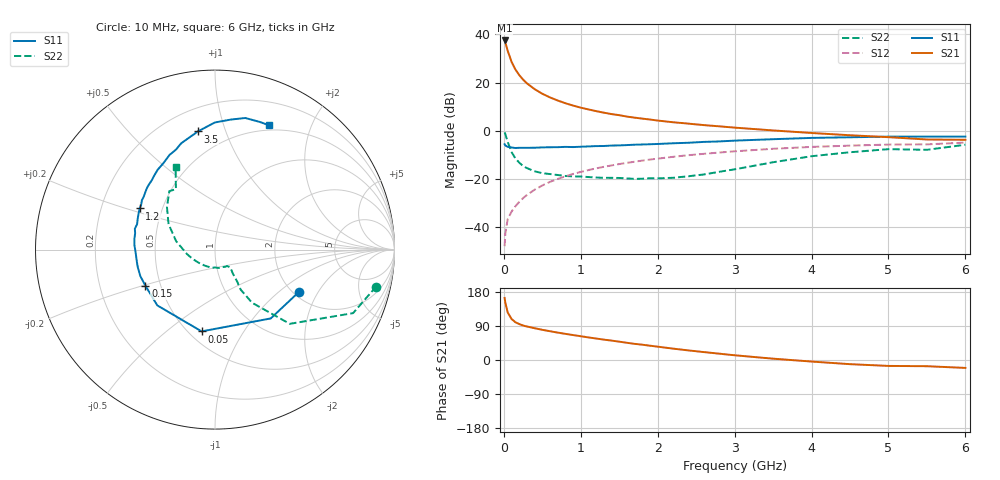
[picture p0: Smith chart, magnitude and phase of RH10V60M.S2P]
! SIEMENS Small Signal Semiconductors
! BFR106
! Si NPN RF Bipolar Junction Transistor in SOT23
! VCE = 10 V  IC = 60 mA
! Common Emitter S-Parameters:  August  1996
# GHz  S  MA  R  50
!  f  S11  S21  S12  S22
! GHz  MAG  ANG  MAG  ANG  MAG  ANG  MAG  ANG
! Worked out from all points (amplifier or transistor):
!   36 points, 10 MHz to 6 GHz, reference 50 ohm
!   highest |S21| = 37.5 dB at 10 MHz (marker M1)
!   |S21| within 3 dB of that: start of sweep to 38.71 MHz
!   unconditionally stable (mu >= 1): 246.6 MHz to 2.323 GHz
!   at 250 MHz: K = 1.00, MAG = 24.3 dB, |S12| = -28.0 dB
!   at 1.4 GHz: K = 1.06, MAG = 9.1 dB, |S12| = -14.4 dB
!   at 6 GHz: K = 0.98, MSG = 0.6 dB, |S12| = -4.9 dB
!   S11 on the Smith chart (normalised r, x): 10 MHz: 2.13, -1.39; 50 MHz: 0.58, -0.67; 150 MHz: 0.41, -0.21; 1.2 GHz: 0.37, +0.22; 3.5 GHz: 0.34, +0.81; 6 GHz: 0.44, +1.43
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0.01  0.5233 -26.9  74.74 163.6  0.004 82.9  0.9213 -12.9
0.02  0.4935 -51.0  67.52 150.8  0.0075 70.4  0.8469 -24.7
0.05  0.4618 -99.3  45.67 125.6  0.0145 60.0  0.587 -44.8
0.1  0.4473 -136.0  27.02 108.2  0.0209 60.7  0.3611 -55.1
0.15  0.4368 -152.5  18.7 99.7  0.0269 62.6  0.2656 -57.3
0.2  0.4415 -160.5  14.31 94.9  0.0332 66.6  0.2173 -55.3
0.25  0.4412 -167.2  11.49 91.0  0.0398 68.5  0.1841 -54.1
0.3  0.4407 -171.2  9.625 88.4  0.0462 69.4  0.1672 -53.4
0.4  0.4426 -178.0  7.291 83.9  0.0595 71.4  0.1436 -50.9
0.5  0.4498 176.7  5.848 79.7  0.0728 71.2  0.1311 -49.2
0.6  0.453 172.6  4.908 76.0  0.0865 71.0  0.1258 -50.1
0.7  0.4543 168.4  4.234 72.3  0.0996 70.7  0.1202 -51.7
0.9  0.4567 161.9  3.32 65.8  0.1264 68.6  0.1125 -54.7
1.1  0.4712 154.5  2.763 59.6  0.1521 66.4  0.109 -62.3
1.2  0.4785 151.4  2.548 56.7  0.165 65.3  0.1065 -65.6
1.6  0.5027 140.6  1.961 45.4  0.2148 60.0  0.1021 -84.0
2.2  0.5476 125.7  1.497 30.0  0.2866 51.9  0.1052 -120.6
2.8  0.5981 111.3  1.232 16.7  0.3518 43.2  0.1401 -161.3
3.5  0.6654 98.2  1.012 3.5  0.421 33.2  0.2211 167.9
4.5  0.7297 83.1  0.804 -11.0  0.4895 18.6  0.3568 138.6
5.5  0.7537 70.6  0.656 -16.4  0.52 8.4  0.4009 122.9
6  0.7555 66.5  0.647 -20.9  0.5661 1.4  0.5104 115.5
